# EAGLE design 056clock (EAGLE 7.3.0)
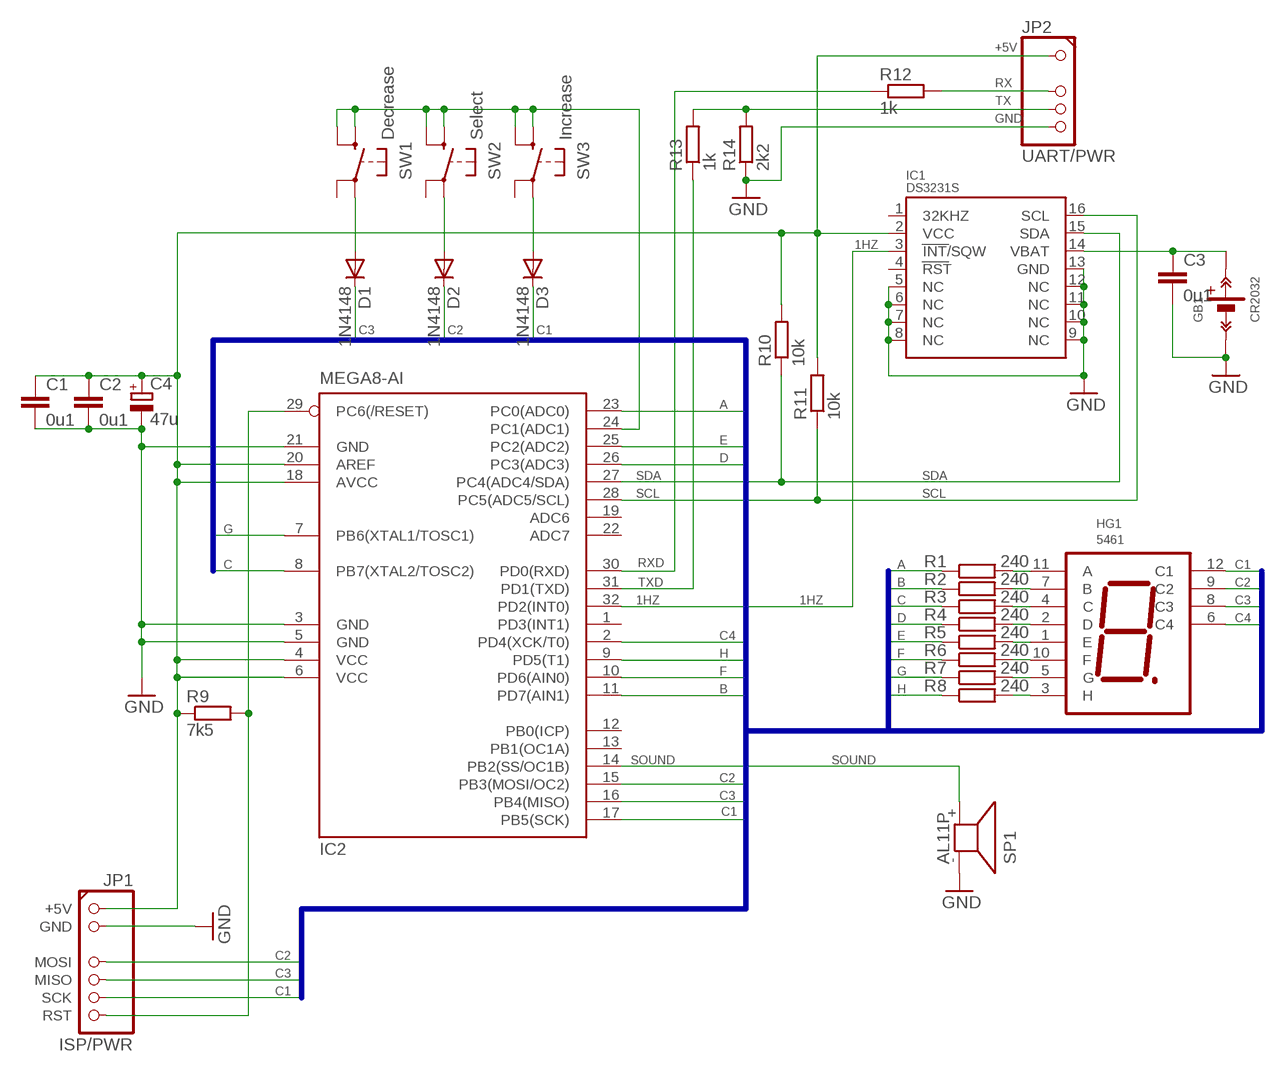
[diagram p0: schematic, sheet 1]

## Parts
C1  0u1  C-EUC1206  [C1206]
C2  0u1  C-EUC1206  [C1206]
C3  0u1  C-EUC1206  [C1206]
C4  47u  CPOL-EUE2.5-6  [E2,5-6]
D1  1N4148  [SOD80-R]
D2  1N4148  [SOD80-R]
D3  1N4148  [SOD80-R]
GB1  CR2032  CR2032_HOLDER/CH224  [CH224-2032]
HG1  5461  4X_7SEG_COMMON_CATHODES/KYX-5461AB  [4X_7SEG_KYX-5461AB]
IC1  DS3231S  [SO16W]
IC2  MEGA8-AI  [TQFP32-08]
JP1  ISP/PWR  CONN1X7(2+4)_ISP+  [1X07_ISP+]
JP2  UART/PWR  CONN1X5(1+3)  [1X05(1+3)]
R1  240  R-EU_R0805  [R0805]
R2  240  R-EU_R0805  [R0805]
R3  240  R-EU_R0805  [R0805]
R4  240  R-EU_R0805  [R0805]
R5  240  R-EU_R0805  [R0805]
R6  240  R-EU_R0805  [R0805]
R7  240  R-EU_R0805  [R0805]
R8  240  R-EU_R0805  [R0805]
R9  7k5  R-EU_R1206  [R1206]
R10  10k  R-EU_R1206  [R1206]
R11  10k  R-EU_R1206  [R1206]
R12  1k  R-EU_R0805  [R0805]
R13  1k  R-EU_R0805  [R0805]
R14  2k2  R-EU_R1206  [R1206]
SP1  AL11P  [AL11P]
SW1  Decrease  TACT_BUTTON  [BUTTON_SMD_4.5X4.5]
SW2  Select  TACT_BUTTON  [BUTTON_SMD_4.5X4.5]
SW3  Increase  TACT_BUTTON  [BUTTON_SMD_4.5X4.5]

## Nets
1HZ: IC1.3(INT/SQW) IC2.32(PD2(INT0))
+5V: C1.1 C2.1 C4.+ IC1.2(VCC) IC2.4(VCC) IC2.6(VCC) IC2.18(AVCC) IC2.20(AREF) JP1.+5V JP2.1 R9.1 R10.2 R11.2
A: IC2.23(PC0(ADC0)) R1.1
B: IC2.11(PD7(AIN1)) R2.1
C: IC2.8(PB7(XTAL2/TOSC2)) R3.1
C1: D3.C HG1.12(C1) IC2.17(PB5(SCK)) JP1.SCK
C2: D2.C HG1.9(C2) IC2.15(PB3(MOSI/OC2)) JP1.MOSI
C3: D1.C HG1.8(C3) IC2.16(PB4(MISO)) JP1.MISO
C4: HG1.6(C4) IC2.2(PD4(XCK/T0))
D: IC2.26(PC3(ADC3)) R4.1
E: IC2.25(PC2(ADC2)) R5.1
F: IC2.10(PD6(AIN0)) R6.1
G: IC2.7(PB6(XTAL1/TOSC1)) R7.1
GND: C1.2 C2.2 C3.2 C4.- GB1.GB- IC1.5(NC) IC1.6(NC) IC1.7(NC) IC1.8(NC) IC1.9(NC) IC1.10(NC) IC1.11(NC) IC1.12(NC) IC1.13(GND) IC2.3(GND) IC2.5(GND) IC2.21(GND) JP1.GND JP2.5 R14.1 SP1.-
H: IC2.9(PD5(T1)) R8.1
N$4: HG1.11(A) R1.2
N$5: HG1.7(B) R2.2
N$6: HG1.4(C) R3.2
N$7: HG1.2(D) R4.2
N$8: HG1.1(E) R5.2
N$9: HG1.10(F) R6.2
N$10: HG1.5(G) R7.2
N$11: HG1.3(H) R8.2
N$14: C3.1 GB1.GB+ IC1.14(VBAT)
N$17: IC2.29(PC6(/RESET)) JP1.RST R9.2
N$20: D1.A SW1.P
N$21: IC2.24(PC1(ADC1)) SW1.S SW1.S@1(S) SW2.S SW2.S@1(S) SW3.S SW3.S@1(S)
N$22: D2.A SW2.P
N$24: D3.A SW3.P
RX: JP2.3 R12.2
RXD: IC2.30(PD0(RXD)) R12.1
SCL: IC1.16(SCL) IC2.28(PC5(ADC5/SCL)) R11.1
SDA: IC1.15(SDA) IC2.27(PC4(ADC4/SDA)) R10.1
SOUND: IC2.14(PB2(SS/OC1B)) SP1.+
TX: JP2.4 R13.2 R14.2
TXD: IC2.31(PD1(TXD)) R13.1
Unconnected: IC1.1(32KHZ) IC1.4(RST) IC2.1(PD3(INT1)) IC2.12(PB0(ICP)) IC2.13(PB1(OC1A)) IC2.19(ADC6) IC2.22(ADC7) SW1.P@1(P) SW2.P@1(P) SW3.P@1(P)

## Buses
A,B,C,D,E,F,G,H,C1,C2,C3,C4

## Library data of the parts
C1-C3 = rcl:C-EU: CAPACITOR, European symbol
C4 = rcl:CPOL-EU: POLARIZED CAPACITOR, European symbol
D1-D3 = diode:1N4148: DIODE
GB1 = !_AndyLib:CR2032_HOLDER
HG1 = !_AndyLib:4X_7SEG_COMMON_CATHODES: LED MODULES
IC1 = !_AndyLib:DS3231S
IC2 = atmel:MEGA8: MICROCONTROLLER 8 Kbytes FLASH, 1 kbytes SRAM, 512 bytes EEPROM, USART, 6-channel 10 bit ADC, 2-channel 8 bit ADC Pin compatible with Atmega48, ATMega88, ATMega168 Source: avr.lbr; MPN: ATMEGA8-16AU; OC_FARNELL: 9171371; OC_NEWARK: 73M8863
JP1 = !_AndyLib:CONN1X7(2+4)_ISP+: PIN HEADER
JP2 = !_AndyLib:CONN1X5(1+3)
R1-R14 = rcl:R-EU_: RESISTOR, European symbol
SP1 = buzzer:AL11P: SPEAKER; OC_FARNELL: unknown; OC_NEWARK: unknown
SW1-SW3 = !_AndyLib:TACT_BUTTON

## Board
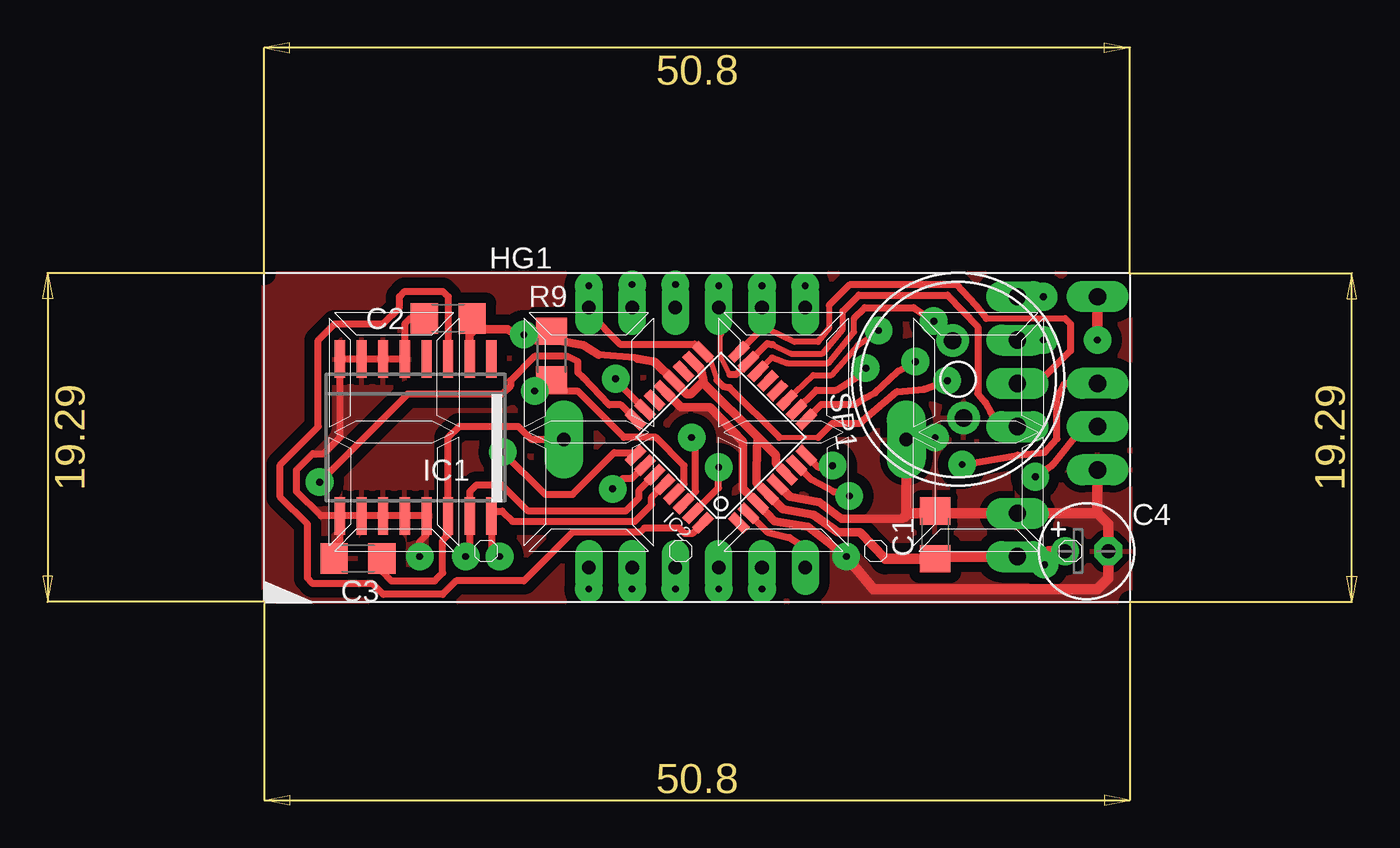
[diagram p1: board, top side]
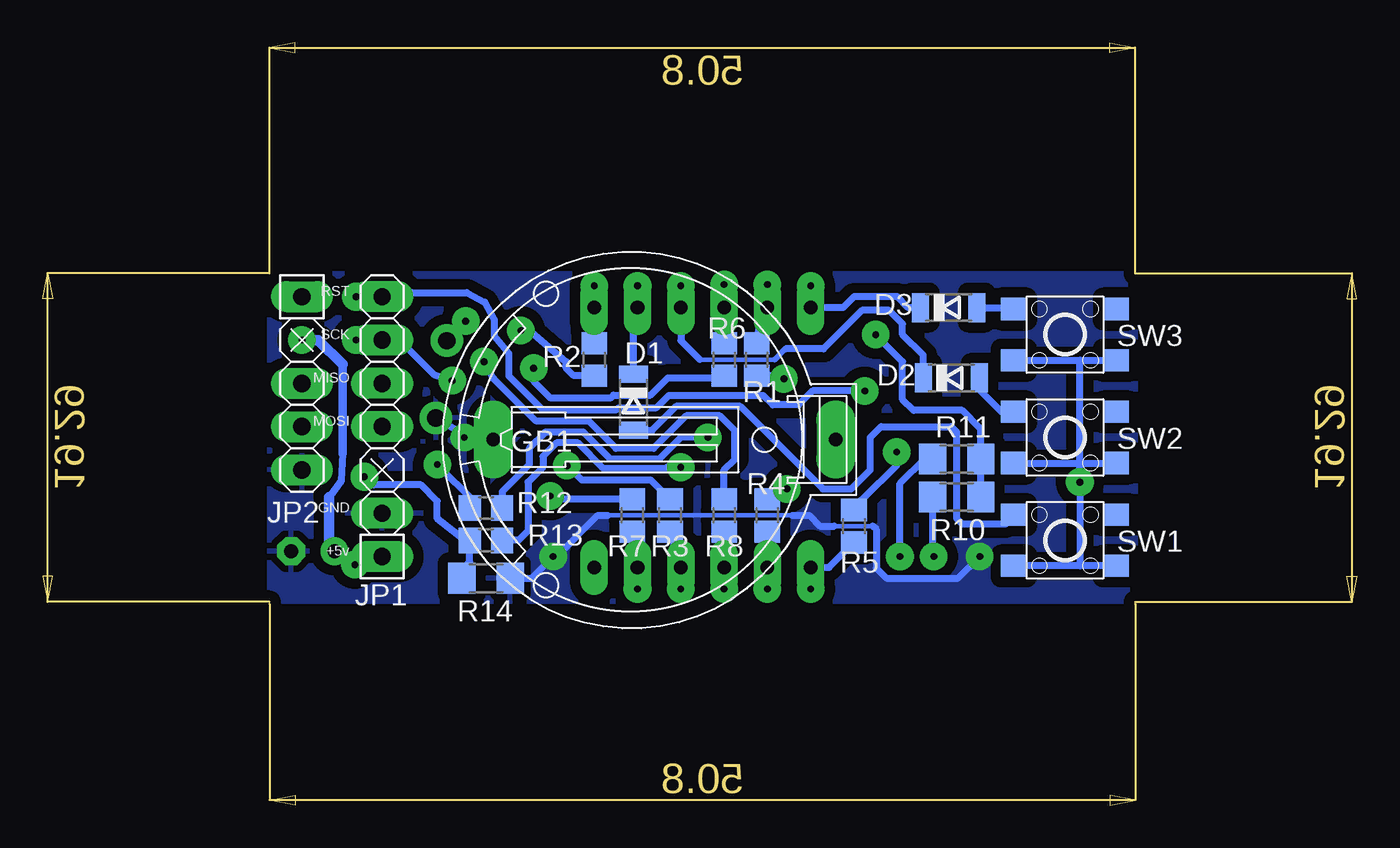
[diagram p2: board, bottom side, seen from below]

Size 77.12 x 44.73 mm. Coordinates in mm from the lower left corner, seen from the top.
Copper layers (1*16): Top 0.035mm / dielectric 1.5mm / Bottom 0.035mm
Design rules "default": minimum track width 12mil, minimum drill 14mil, track to track 8mil, track to pad 8mil, pad to pad 8mil, via to via 8mil, smd to smd 8mil, copper to edge 20mil, drill to drill 30mil, minimum pad ring 16mil, minimum via ring 24mil, stop-mask expansion 4mil, vias tented up to drill 0mil, thermal gap 16mil

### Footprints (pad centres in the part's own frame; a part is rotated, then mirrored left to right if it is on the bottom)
C1206 = smd 1.6 x 1.8: 1 -1.4,0; 2 1.4,0
E2,5-6 = drill 0.813 pad 1.6: + -1.27,0 | drill 0.813 pad 1.6 octagon: - 1.27,0
SOD80-R = smd 1 x 1.7: A 1.65,0; C -1.65,0
CH224-2032 = drill 0.8 pad 2.3 long: GB+ -12.05,0; GB- 8.05,0
4X_7SEG_KYX-5461AB = drill 0.8 long: 1 -6.35,-7.62; 2 -3.81,-7.62; 3 -1.27,-7.62; 4 1.27,-7.62; 5 3.81,-7.62; 6 6.35,-7.62; 7 6.35,7.62; 8 3.81,7.62; 9 1.27,7.62; 10 -1.27,7.62; 11 -3.81,7.62; 12 -6.35,7.62
SO16W = smd 0.6 x 2.2: 1 -4.445,-4.6; 2 -3.175,-4.6; 3 -1.905,-4.6; 4 -0.635,-4.6; 5 0.635,-4.6; 6 1.905,-4.6; 7 3.175,-4.6; 8 4.445,-4.6; 9 4.445,4.6; 10 3.175,4.6; 11 1.905,4.6; 12 0.635,4.6; 13 -0.635,4.6; 14 -1.905,4.6; 15 -3.175,4.6; 16 -4.445,4.6
TQFP32-08 = smd 1.27 x 0.559: 1 -4.293,2.8; 2 -4.293,2; 3 -4.293,1.2; 4 -4.293,0.4; 5 -4.293,-0.4; 6 -4.293,-1.2; 7 -4.293,-2; 8 -4.293,-2.8; 17 4.293,-2.8; 18 4.293,-2; 19 4.293,-1.2; 20 4.293,-0.4; 21 4.293,0.4; 22 4.293,1.2; 23 4.293,2; 24 4.293,2.8 | smd 0.559 x 1.27: 9 -2.8,-4.293; 10 -2,-4.293; 11 -1.2,-4.293; 12 -0.4,-4.293; 13 0.4,-4.293; 14 1.2,-4.293; 15 2,-4.293; 16 2.8,-4.293; 25 2.8,4.293; 26 2,4.293; 27 1.2,4.293; 28 0.4,4.293; 29 -0.4,4.293; 30 -1.2,4.293; 31 -2,4.293; 32 -2.8,4.293
1X07_ISP+ = drill 1.016 long: +5V -7.62,0; GND -5.08,0; MISO 2.54,0; MOSI 0,0; RST 7.62,0; SCK 5.08,0
1X05(1+3) = drill 1.016 long: 1 -5.08,0; 3 0,0; 4 2.54,0; 5 5.08,0
R0805 = smd 1.3 x 1.5: 1 -0.95,0; 2 0.95,0
R1206 = smd 1.6 x 1.803: 1 -1.422,0; 2 1.422,0
AL11P = drill 1.016 pad 1.905: + 2.286,0; - -2.286,0
BUTTON_SMD_4.5X4.5 = smd 1.5 x 1.3: P -3,1.5; P@1 3,1.5; S -3,-1.5; S@1 3,-1.5

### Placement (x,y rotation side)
C1  52.37,15.86 90 top
C2  23.79,28.56 180 top
C3  18.51,14.48 180 top
C4  61.26,14.91 0 top
D1  42.45,23.64 270 bottom
D2  23.79,25.07 0 bottom
D3  23.95,29.19 0 bottom
GB1  42.62,21.45 180 bottom
HG1  38.4,21.57 0 top
IC1  21.89,21.57 180 top
IC2  39.8,21.57 135 top
JP1  57.2,22.21 90 bottom
JP2  61.9,24.75 270 bottom
R1  35.22,26.14 90 bottom
R2  44.75,26.14 90 bottom
R3  40.31,17 270 bottom
R4  34.59,17 270 bottom
R5  29.51,16.37 270 bottom
R6  37.13,26.14 90 bottom
R7  42.53,17 270 bottom
R8  37.13,17 270 bottom
R9  29.86,26.38 270 top
R10  23.48,18.08 0 bottom
R11  23.48,20.3 0 bottom
R12  51.1,17.45 180 bottom
R13  51.1,15.54 180 bottom
R14  51.1,13.32 180 bottom
SP1  53.72,24.99 98 top
SW1  17.13,15.54 0 bottom
SW2  17.13,21.57 0 bottom
SW3  17.13,27.61 0 bottom

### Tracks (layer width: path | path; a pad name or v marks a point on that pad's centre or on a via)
1HZ
  Top 0.406: IC2.32 38.12,15.94 37.69,15.94 37.37,16.25 35.3,16.25 35.07,16.02 31.1,16.02 28.24,13.16 24.27,13.16 23.48,12.36 19.98,12.36 19.35,13 15.86,13 15.54,13.32 15.54,16.49 13.95,18.08 13.95,19.99 16.18,22.21 16.18,27.29 17.13,28.24 19.98,28.24 20.94,29.19 20.94,29.83 21.25,30.14 23.48,30.14 23.79,29.83 IC1.3
+5V  (via drill 0.4)
  Top 0.406: 34.91,26.18 34.75,26.26 32.61,26.41 | 25.38,27.92 25.2,27.74 25.07,27.6 | 38.78,24.76 38.78,24.87 | v28.24,27.6 28.24,27.29 | 52.5,14.59 C1.1 | R9.1 29.86,27.57 30.14,27.29
  Top 0.508: IC2.6 43.02,20.05 43.02,20.53 41.93,21.61 | IC2.18 38.62,25.58 38.78,24.87 38.02,24.11 37.82,24.11 IC2.20 35.92,26.02 34.91,26.18 | 32.61,26.41 31.73,26.97 30.14,27.29 28.24,27.29 27.29,27.92 25.38,27.92 | 25.07,27.6 IC1.2 | C2.1 25.2,27.74 | 49.45,14.46 47.97,16.02 46.66,16.02 45.23,17.05 43.44,17.37 IC2.4 41.89,18.91 41.89,19.67 41.93,21.61 | 41.93,21.61 38.78,24.76
  Top 0.61: 52.5,14.59 JP1.+5V 58.72,14.59 | C1.1 49.45,14.46 | C4.+ 59.04,14.91 58.72,14.59 | v58.8,14.11 58.72,14.59 | v61.9,27.29 JP2.1
  Bottom 0.406: R10.2 R11.2 22.06,22.06 23.16,23.16 26.02,23.16 26.65,23.8 26.65,26.02 v28.24,27.6 | 59.51,20.62 59.59,19.03 60.31,18.08 | C4.+ 59.67,14.91
  Bottom 0.508: 59.51,25.86 59.51,20.62
  Bottom 0.61: 59.51,25.86 60.94,27.29 v61.9,27.29 | 60.31,18.08 60.31,15.22 C4.+ | 59.67,14.91 v58.8,14.11
A  (via drill 0.4)
  Top 0.406: IC2.23 33.79,24.75 33.81,24.83 v33.62,25.02
  Bottom 0.406: v33.62,25.02 33.81,25.19 R1.1
B  (via drill 0.4)
  Top 0.356: IC2.11 45.22,25.22 46.29,25.22 47.83,26.99 48.53,27.45
  Top 0.406: 48.53,27.45 v49.05,27.84
  Bottom 0.406: R2.1 45.96,25.19 46.4,25.64 46.4,26.02 48.47,27.76 v49.05,27.84
C  (via drill 0.4)
  Top 0.406: IC2.8 45.5,19.83 46.26,19.83 v46.35,19.92
  Bottom 0.406: 40.62,18.14 R3.1 41.44,19.08 45.48,19.08 45.84,19.45 v46.35,19.92
C1  (via drill 0.4)
  Top 0.305: 39.16,26.17 39.56,24.94 | 43.23,21.57 45.51,21.57
  Top 0.406: HG1.12 32.05,28.88 33.88,27.05 38.28,27.05 IC2.17 39.16,26.17 | 39.56,24.94 39.92,24.57 40.31,24.49 43.23,21.57 | 45.51,21.57 46.34,22.4 47.96,22.4 50.13,24.26 51.72,24.41 v53.08,24.91
  Bottom 0.406: D3.C 26.34,29.19 26.97,29.83 29.51,29.83 30.14,29.19 HG1.12 | v53.08,24.91 54.12,25.22 56.18,27.29 JP1.SCK
C2
  Top 0.305: 40.31,25.26 39.79,26.33 39.79,27.65
  Top 0.356: 42.83,27.02 43.91,26.49 45.77,26.49 46.96,27.92 46.96,28.99
  Top 0.406: HG1.9 39.67,27.77 39.79,27.65 | 40.31,25.26 40.69,25.26 41.42,25.99 IC2.15 41.45,26.02 42.53,27.1 42.83,27.02 | 46.96,28.99 47.89,29.92 53.1,29.92 54.88,28.07 54.88,24.14 55.32,23.62 55.64,23.03 56.15,22.21 JP1.MOSI
  Bottom 0.254: 34.15,26.14 38.56,26.14
  Bottom 0.356: 33.52,26.77 34.15,26.14
  Bottom 0.406: D2.C 25.45,26.4 26.65,27.6 26.65,28.24 27.45,29.03 29.03,29.03 31.3,26.77 33.52,26.77 | HG1.9 39.67,27.25 38.56,26.14
C3
  Top 0.356: 46.15,29.32 46.15,27.99 45.5,27.18 44.13,27.18 42.59,27.92 | 55.37,28.56 59.99,28.56
  Top 0.406: HG1.8 42.21,27.95 | 42.21,27.95 IC2.16 | 46.15,29.32 47.35,30.53 53.64,30.53 54.77,29.32 55.37,28.56 | 42.59,27.92 42.23,27.92 42.21,27.95 | 59.99,28.56 60.31,28.24 60.31,26.65 58.4,24.75 JP1.MISO
  Bottom 0.406: D1.C 42.45,27.68 42.21,27.92 HG1.8
C4
  Top 0.406: IC2.2 42.53,16.02 43.83,15.7 44.75,15.1 HG1.6
D  (via drill 0.4)
  Top 0.406: IC2.26 34.56,19.16 34.05,19.16 v33.45,18.56
  Bottom 0.406: R4.1 34.08,17.95 v33.45,18.56
E  (via drill 0.4)
  Top 0.406: IC2.25 34.61,20.68 33.54,20.68 31.1,18.24 29.49,18.24 v27,20.72
  Bottom 0.406: 29.19,17.41 R5.1 29,17.95 27,19.95 v27,20.72
F  (via drill 0.4)
  Top 0.406: v48.31,25.64 47.86,25.16 46.58,24.35 45.4,24.35 IC2.10
  Bottom 0.406: R6.1 37.26,25.07 40.43,25.06 41.45,24.05 43.62,24.05 43.8,23.87 47.31,23.87 48.31,24.87 v48.31,25.64
G  (via drill 0.4)
  Top 0.406: v47.34,18.14 46.43,18.38 45.1,19.1 IC2.7
  Bottom 0.406: R7.1 47.06,17.95 v47.34,18.14
GND  (via drill 0.4)
  Top 0.406: 50.59,16.94 50.47,16.81 | 47.1,14.65 v47.16,14.59 | 50.67,17.21 50.91,17.13 | IC1.9 IC1.10 IC1.11 IC1.12 IC1.13 22.53,15.86 22.13,15.46 v22.13,14.59 | C2.2 21.57,28.56 21.25,28.24 IC1.5 IC1.6 IC1.7 IC1.8 17.45,21.57 16.49,20.62 15.86,20.62 14.91,19.67 14.91,18.4 16.33,16.97 IC1.9 | 52.5,17.13 C1.2 52.37,17.13 | C3.2 17.11,15.2 17.45,15.54 IC1.9 | v52.37,21.57 50.8,21.57 GB1.GB-
  Top 0.508: IC2.21 37.45,23.36 39.16,23.36 41.1,21.33 41.1,18.57 IC2.3 42.94,16.65 44.91,16.33 46.62,15.02 47.1,14.65 | 50.47,16.81 46.86,16.81 45.58,17.78 43.84,18.1 IC2.5
  Top 0.61: 52.37,17.13 50.91,17.13 50.59,16.94 | GB1.GB- 50.67,17.21 | 52.5,17.13 JP1.GND 61.9,17.13 | v47.16,14.59 48.75,12.68 61.9,12.68 62.53,13.32 C4.- 62.53,16.49 61.9,17.13 | JP2.5 61.9,17.13
  Bottom 0.254: 43.96,17.01 33.12,17.01 | 30.66,16.37 28.4,16.37
  Bottom 0.406: 43.96,17.01 44.55,17.01 46.97,14.59 v47.16,14.59 48.43,13.32 R14.1 | 33.12,17.01 32.13,17.01 31.49,16.37 30.66,16.37 | 28.4,16.37 28.2,16.17 28.2,13.91 27.61,13.32 23.4,13.32 v22.13,14.59 | SP1.- 52.77,21.97 v52.37,21.57
  pour Top (isolate 0.61): 63.8,31.22 63.8,11.93 13,11.93 13,31.22
  pour Bottom (isolate 0.61): 13,31.22 13,11.93 63.8,11.93 63.8,31.22
H  (via drill 0.4)
  Top 0.406: v51.21,26.02 50.2,25.46 48.85,24.19 48.23,23.87 47.7,23.51 45.69,23.51 IC2.9
  Bottom 0.406: R8.1 37.13,19.67 36.5,20.3 36.5,21.95 37.38,22.84 39.35,22.84 41.26,20.94 43.48,20.94 45.07,22.53 48.16,22.53 50.66,25.02 v51.21,26.02
N$4  (via drill 0.4)
  Bottom 0.406: R1.2 v34.59,30.54 HG1.11
N$5
  Bottom 0.406: HG1.7 R2.2
N$6
  Bottom 0.406: R3.2 HG1.4
N$7
  Bottom 0.406: R4.2 HG1.2
N$8
  Bottom 0.406: HG1.1 30.97,13.95 R5.2
N$9  (via drill 0.4)
  Bottom 0.406: R6.2 v37.13,30.54 HG1.10
N$10
  Bottom 0.406: R7.2 HG1.5
N$11
  Bottom 0.406: R8.2 HG1.3
N$12  (via drill 0.4)
  other vias: 32.05,12.68
N$13  (via drill 0.4)
  other vias: 34.59,12.68
N$14
  Top 0.406: GB1.GB+ 28.68,21.45 27.92,22.21 24.43,22.21 23.79,21.57 IC1.14 23.79,15.86 23.48,15.54 23.48,13.63 23,13.16 20.46,13.16 19.91,13.71 C3.1
N$15  (via drill 0.4)
  other vias: 37.13,12.68
N$16  (via drill 0.4)
  other vias: 39.67,12.68
N$17  (via drill 0.4)
  Top 0.406: IC2.29 37.64,18.85 37.64,19.92 35.99,21.57 34.11,21.57 31.38,24.3 29.83,24.3 | v28.88,24.3 29.83,24.3 | R9.2 29.86,24.33 29.83,24.3
  Bottom 0.406: v28.88,24.3 31.94,24.3 32.76,23.48 34.27,23.48 34.83,24.03 40.38,24.03 41.13,23.29 43.35,23.29 43.43,23.21 47.78,23.21 49.75,25.18 49.75,26.49 50.62,27.53 50.62,28.48 51.18,29.51 52.21,30.07 55.47,30.07 55.86,29.83 JP1.RST
N$18  (via drill 0.4)
  other vias: 42.21,12.68
N$19  (via drill 0.4)
  other vias: 44.75,30.46
N$20
  Bottom 0.406: D1.A 41.35,21.99 39.94,23.4 36.18,23.4 31.34,18.56 29.67,18.56 28.56,19.67 28.56,21.57 27.92,22.21 23.79,22.21 23.48,21.89 23.48,16.81 23.16,16.49 20.62,16.49 20.13,16.99 SW1.P
N$21  (via drill 0.4)
  Top 0.406: IC2.24 33.93,23.48 33.24,23.48 31.73,25.06 31.42,25.38 31.42,26.02 30.78,26.34 28.88,26.34 27.45,24.91 27.45,24.59 26.97,24.11 21.41,24.11 v16.25,18.95
  Bottom 0.406: SW2.S 20.04,19.99 20.04,20.07 16.25,20.07 | 16.25,14.04 v16.25,18.95 16.25,20.07 | 16.25,14.04 SW1.S | 16.25,20.07 16.25,26.1 | 16.25,26.1 SW3.S@1 | 16.25,20.07 SW2.S@1 | SW1.S@1 16.25,14.04 | SW3.S 16.25,26.1
N$22
  Bottom 0.406: SW2.P 20.85,23.07 22.14,24.37 D2.A
N$23  (via drill 0.4)
  other vias: 58.72,27.29
N$24
  Bottom 0.406: D3.A 20.62,29.19 20.13,29.02 SW3.P
N$26  (via drill 0.4)
  other vias: 58.72,29.83
N$28  (via drill 0.4)
  other vias: 32.05,30.46
N$30  (via drill 0.4)
  other vias: 39.67,30.46
N$31  (via drill 0.4)
  other vias: 42.21,30.46
RX  (via drill 0.4)
  Top 0.406: v53.96,19.99 57.21,20.54 58.8,20.7 59.51,21.49 59.51,23.87 59.99,24.75 JP2.3
  Bottom 0.406: R12.2 51.73,17.76 v53.96,19.99
RXD  (via drill 0.4)
  Top 0.406: IC2.30 38.32,18.4 38.32,20.94 38.08,21.18 v38.08,21.57
  Bottom 0.406: v38.08,21.57 39.67,21.57 40.94,20.3 43.8,20.3 45.39,21.89 47.61,21.89 48.56,20.94 48.56,19.99 50.15,18.4 50.15,17.77 R12.1
SCL  (via drill 0.4)
  Top 0.406: IC2.28 35.73,18.07 35.73,17.64 34.75,16.65 27.57,16.65 26.97,17.25 26.62,17.25 IC1.16 26.34,14.91 v26.81,14.59
  Bottom 0.406: v26.81,14.59 26.81,18.87 25.38,20.3 R11.1
SDA  (via drill 0.4)
  Top 0.406: IC2.27 34.97,18.44 34.97,18.02 34.21,17.25 28.49,17.25 26.97,18.78 25.45,18.78 25.07,18.4 IC1.15 25.07,15.06 v24.83,14.59
  Bottom 0.406: v24.83,14.59 24.83,14.91 24.9,15.06 R10.1
SOUND  (via drill 0.4)
  Top 0.356: IC2.14 42.78,26.26 42.84,26.26 43.72,25.94 46.1,25.94 47.61,27.76 47.61,28.56
  Top 0.406: 47.61,28.56 48.24,29.19 51.1,29.19 v52.29,28.4
  Bottom 0.406: v52.29,28.4 53.08,27.55 SP1.+
TX  (via drill 0.4)
  Top 0.406: v58.24,19.27 59.28,19.99 61.02,22.13 JP2.4
  Bottom 0.406: R14.2 52.52,13.8 52.05,14.27 R13.2 52.37,15.54 53.96,16.81 53.96,17.84 54.91,18.79 57.69,18.79 v58.24,19.27
TXD  (via drill 0.4)
  Top 0.406: IC2.31 39.67,18.62 v39.67,19.83
  Bottom 0.406: v39.67,19.83 40.46,19.83 40.54,19.75 44.19,19.75 45.7,21.25 46.97,21.25 47.77,20.46 47.77,19.83 48.64,18.95 48.64,16.1 49.2,15.54 R13.1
